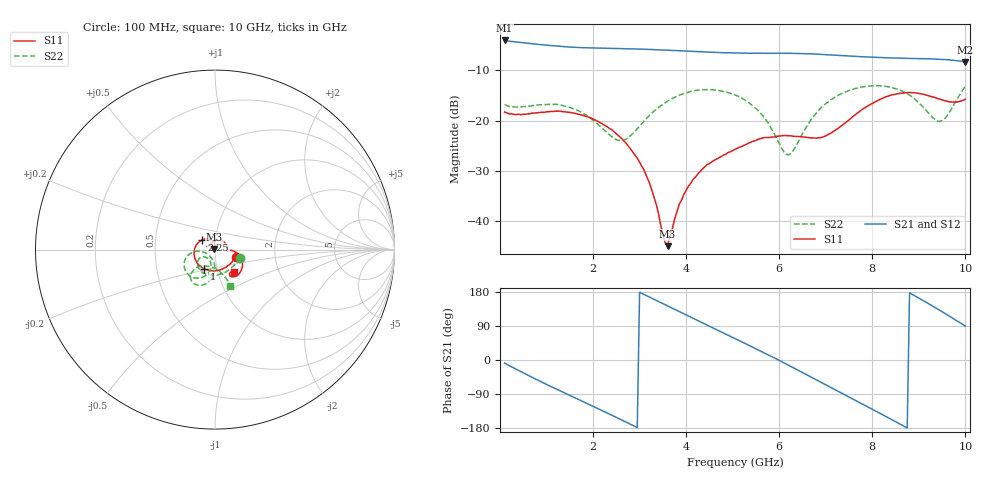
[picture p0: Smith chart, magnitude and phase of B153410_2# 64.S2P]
!  2-Port S-parameters saved by WinCal
! VAR MeasName=S-Parameters (CALIBRATED_DATA) read from VNA (N5245A)
! VAR MeasDate=2016-12-23 10:03:00
! VAR NAME=B153410_2# 64
! VAR FILENAME=B153410_2# 64.S2P
! VAR DATE=2016-12-23 10:03:00
! VAR PHYS_PORTS=1,2
# Hz S DB R 50
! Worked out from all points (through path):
!   199 points, 100 MHz to 10 GHz, reference 50 ohm
!   highest |S21| = -4.03 dB at 100 MHz (marker M1); lowest = -8.3 dB at 10 GHz (marker M2)
!   group delay of S21, straight-line fit = 171 ps
!   lowest |S11| = -45.0 dB at 3.6 GHz (marker M3), VSWR 1.01, Z = 49.6 + j0.39 ohm
!   |S11| at or under -10 dB: start of sweep to end of sweep
!   |S22| runs from -26.8 to -13.0 dB; largest |S21 - S12| = 0.0038
!   S11 on the Smith chart (normalised r, x): 100 MHz: 1.26, -0.10; 1 GHz: 0.86, -0.19; 2.25 GHz: 0.86, +0.09; 10 GHz: 1.20, -0.30
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1e8  -18.26 -19.5  -4.03 -8.0  -4.05 -8.0  -16.81 -18.1
5.5e8  -18.70 -75.8  -4.55 -37.1  -4.57 -37.0  -17.18 -68.3
1e9  -18.23 -120.5  -4.97 -64.4  -4.96 -64.3  -16.78 -104.3
1.75e9  -18.85 179.5  -5.46 -107.9  -5.45 -108.0  -18.34 -143.9
2.25e9  -20.92 143.8  -5.59 -136.7  -5.59 -136.8  -21.92 -149.6
2.6e9  -23.41 119.7  -5.65 -157.4  -5.66 -157.4  -23.95 -129.3
2.95e9  -27.46 96.5  -5.73 -178.3  -5.74 -178.3  -21.61 -105.9
3.2e9  -32.08 84.3  -5.81 166.7  -5.81 166.7  -19.06 -103.3
3.4e9  -38.20 81.6  -5.89 154.6  -5.89 154.7  -17.41 -105.7
3.6e9  -44.95 135.9  -5.96 142.7  -5.96 142.7  -16.12 -110.7
3.85e9  -36.66 176.5  -6.08 127.6  -6.09 127.7  -14.93 -118.1
4.15e9  -31.65 161.9  -6.20 109.8  -6.21 109.9  -14.07 -128.3
5.05e9  -25.70 82.0  -6.52 56.5  -6.53 56.7  -14.87 -159.6
5.65e9  -23.41 33.6  -6.59 20.5  -6.59 20.6  -19.03 -174.9
6.15e9  -22.95 4.9  -6.58 -10.6  -6.59 -10.5  -26.68 -143.5
6.3e9  -23.09 -1.8  -6.60 -20.3  -6.62 -20.1  -25.96 -114.1
6.7e9  -23.41 -8.8  -6.70 -46.0  -6.72 -45.9  -19.60 -90.4
7.5e9  -19.83 -3.9  -7.09 -97.7  -7.12 -97.6  -13.98 -106.0
8.35e9  -15.07 -29.9  -7.51 -152.9  -7.49 -152.4  -13.26 -127.4
8.9e9  -14.43 -50.1  -7.64 170.4  -7.61 170.6  -15.60 -136.4
9.45e9  -15.71 -60.4  -7.78 131.1  -7.78 131.3  -20.14 -103.7
1e10  -15.70 -48.6  -8.30 89.4  -8.31 89.7  -13.09 -67.4
